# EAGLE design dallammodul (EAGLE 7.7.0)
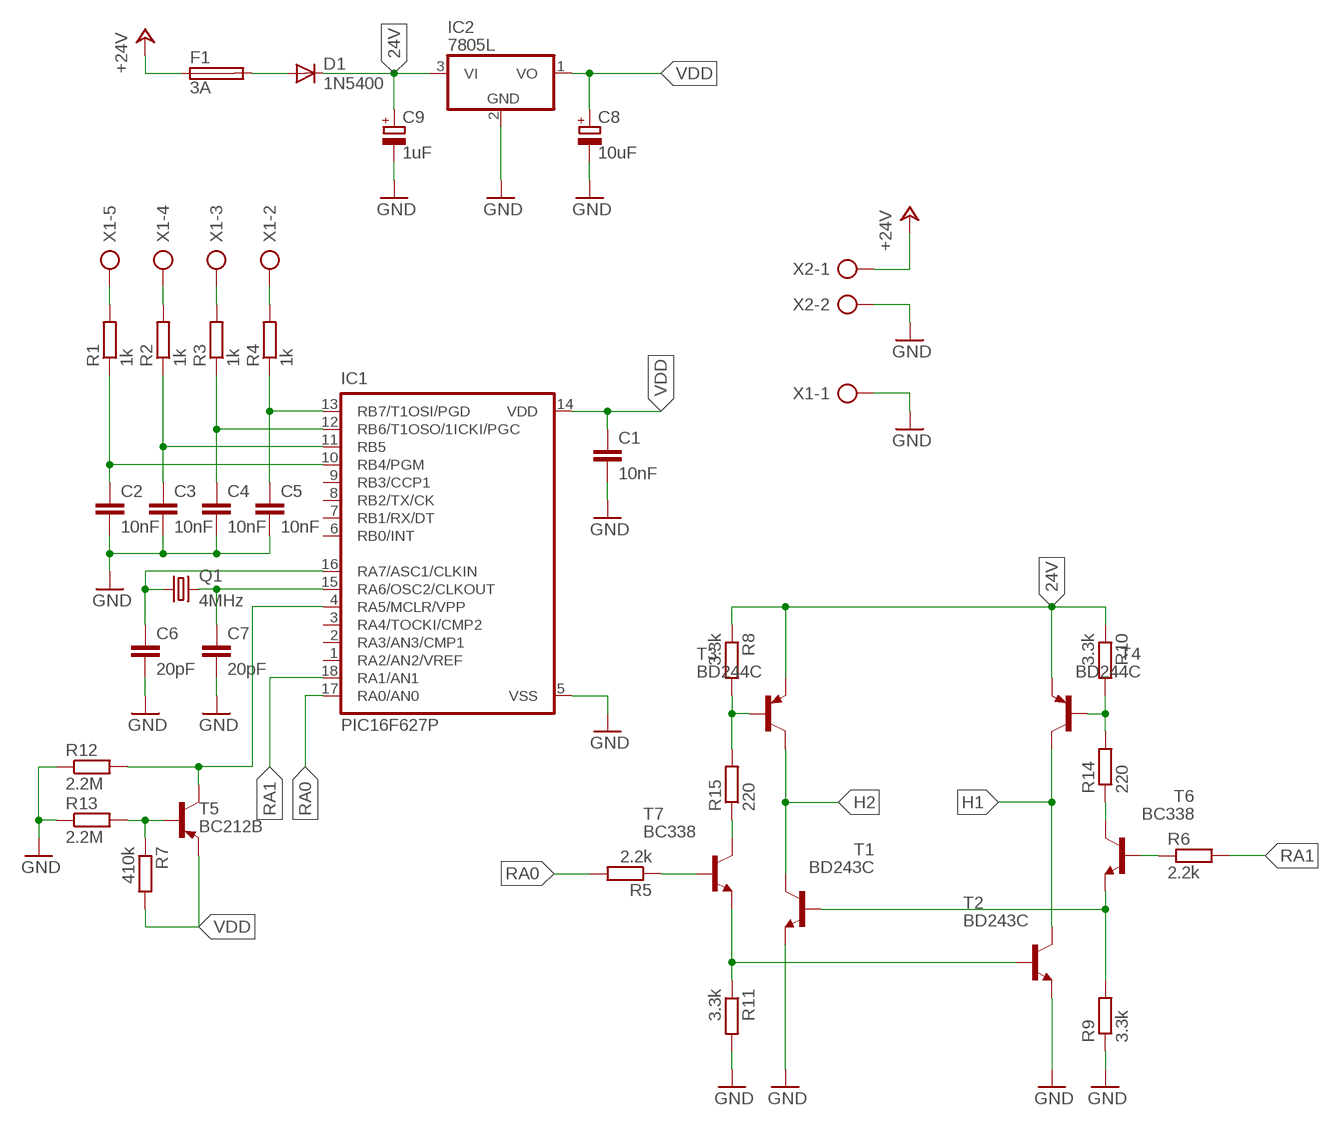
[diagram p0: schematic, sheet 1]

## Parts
C1  10nF  C-EU050-024X044  [C050-024X044]
C2  10nF  C-EU050-024X044  [C050-024X044]
C3  10nF  C-EU050-024X044  [C050-024X044]
C4  10nF  C-EU050-024X044  [C050-024X044]
C5  10nF  C-EU050-024X044  [C050-024X044]
C6  20pF  C-EU050-024X044  [C050-024X044]
C7  20pF  C-EU050-024X044  [C050-024X044]
C8  10uF  CPOL-EUE2-5  [E2-5]
C9  1uF  CPOL-EUE2-5  [E2-5]
D1  1N5400  [DO201-15]
F1  3A  GSH15  [GSH15]
IC1  PIC16F627P  [DIL18]
IC2  7805L  [TO92]
Q1  4MHz  CRYSTALHC18U-V  [HC18U-V]
R1  1k  R-EU_0207/10  [0207/10]
R2  1k  R-EU_0207/10  [0207/10]
R3  1k  R-EU_0207/10  [0207/10]
R4  1k  R-EU_0207/10  [0207/10]
R5  2.2k  R-EU_0207/10  [0207/10]
R6  2.2k  R-EU_0207/10  [0207/10]
R7  410k  R-EU_0207/10  [0207/10]
R8  3.3k  R-EU_0207/10  [0207/10]
R9  3.3k  R-EU_0207/10  [0207/10]
R10  3.3k  R-EU_0207/10  [0207/10]
R11  3.3k  R-EU_0207/10  [0207/10]
R12  2.2M  R-EU_0309/10  [0309/10]
R13  2.2M  R-EU_0309/10  [0309/10]
R14  220  R-EU_0411/15  [0411/15]
R15  220  R-EU_0411/15  [0411/15]
T1  BD243C  -NPN-TO220V  [TO220V]
T2  BD243C  -NPN-TO220V  [TO220V]
T3  BD244C  -PNP-TO220V  [TO220V]
T4  BD244C  -PNP-TO220V  [TO220V]
T5  BC212B  -PNP-TO92L  [TO92L]
T6  BC338  -NPN-TO92L  [TO92L]
T7  BC338  -NPN-TO92L  [TO92L]
X1  AK300/5  [AK300/5]
X2  AK300/2  [AK300/2]

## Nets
24V: C9.+ D1.C IC2.3(VI) R8.1 R10.1 T3.3(E) T4.3(E)
+24V: F1.1 X2.1
GND: C1.2 C2.2 C3.2 C4.2 C5.2 C6.2 C7.2 C8.- C9.- IC1.5(VSS) IC2.2(GND) R9.1 R11.2 R12.1 R13.1 T1.3(E) T2.3(E) X1.1 X2.2
H1: T2.2(C) T4.2(C)
H2: T1.2(C) T3.2(C)
N$1: C6.1 IC1.16(RA7/ASC1/CLKIN) Q1.1
N$2: C7.1 IC1.15(RA6/OSC2/CLKOUT) Q1.2
N$3: C2.1 IC1.10(RB4/PGM) R1.1
N$4: C3.1 IC1.11(RB5) R2.1
N$5: R5.1 T7.2(B)
N$6: C4.1 IC1.12(RB6/T1OSO/1ICKI/PGC) R3.1
N$7: C5.1 IC1.13(RB7/T1OSI/PGD) R4.1
N$8: R4.2 X1.2
N$9: R3.2 X1.3
N$10: R2.2 X1.4
N$11: R1.2 X1.5
N$14: D1.A F1.2
N$15: R8.2 R15.2 T3.1(B)
N$16: R10.2 R14.2 T4.1(B)
N$17: R7.1 R13.2 T5.2(B)
N$18: R15.1 T7.3(C)
N$19: R6.1 T6.2(B)
N$20: R11.1 T2.1(B) T7.1(E)
N$22: R9.2 T1.1(B) T6.1(E)
N$23: R14.1 T6.3(C)
RA0: IC1.17(RA0/AN0) R5.2
RA1: IC1.18(RA1/AN1) R6.2
RA5: IC1.4(RA5/MCLR/VPP) R12.2 T5.3(C)
VDD: C1.1 C8.+ IC1.14(VDD) IC2.1(VO) R7.2 T5.1(E)
Unconnected: IC1.1(RA2/AN2/VREF) IC1.2(RA3/AN3/CMP1) IC1.3(RA4/TOCKI/CMP2) IC1.6(RB0/INT) IC1.7(RB1/RX/DT) IC1.8(RB2/TX/CK) IC1.9(RB3/CCP1)

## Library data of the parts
C1-C7 = rcl:C-EU: CAPACITOR, European symbol
C8 C9 = rcl:CPOL-EU: POLARIZED CAPACITOR, European symbol
D1 = diode:1N5400: DIODE
F1 = fuse:GSH15: FUSE HOLDER; MPN: 64900001039; OC_FARNELL: 1271673; OC_NEWARK: 02P0318
IC1 = microchip:PIC16*F62: FLASH-Based 8-Bit CMOS Microcontroller Source: http://ww1.microchip.com/downloads/en/DeviceDoc/40300C.pdf; MF: MICROCHIP; MPN: PIC16F627-20I/P; OC_FARNELL: 1084298; OC_NEWARK: 23C4967
IC2 = 78:78*: Positive VOLTAGE REGULATOR Source: http://cache.national.com/ds/LM/LM78L05.pdf http://www.fairchildsemi.com/ds/LM/LM7805.pdf
Q1 = crystal:CRYSTAL: CRYSTAL; OC_FARNELL: unknown; OC_NEWARK: unknown
R1-R15 = rcl:R-EU_: RESISTOR, European symbol
T1 T2 T6 T7 = transistor:*-NPN-: NPN Transistror BF959 corrected 2008.03.06
T3-T5 = transistor:*-PNP-: PNP Transistror
X1 = con-ptr500:AK300/5: CONNECTOR; OC_FARNELL: unknown; OC_NEWARK: unknown
X2 = con-ptr500:AK300/2: CONNECTOR; OC_FARNELL: unknown; OC_NEWARK: unknown

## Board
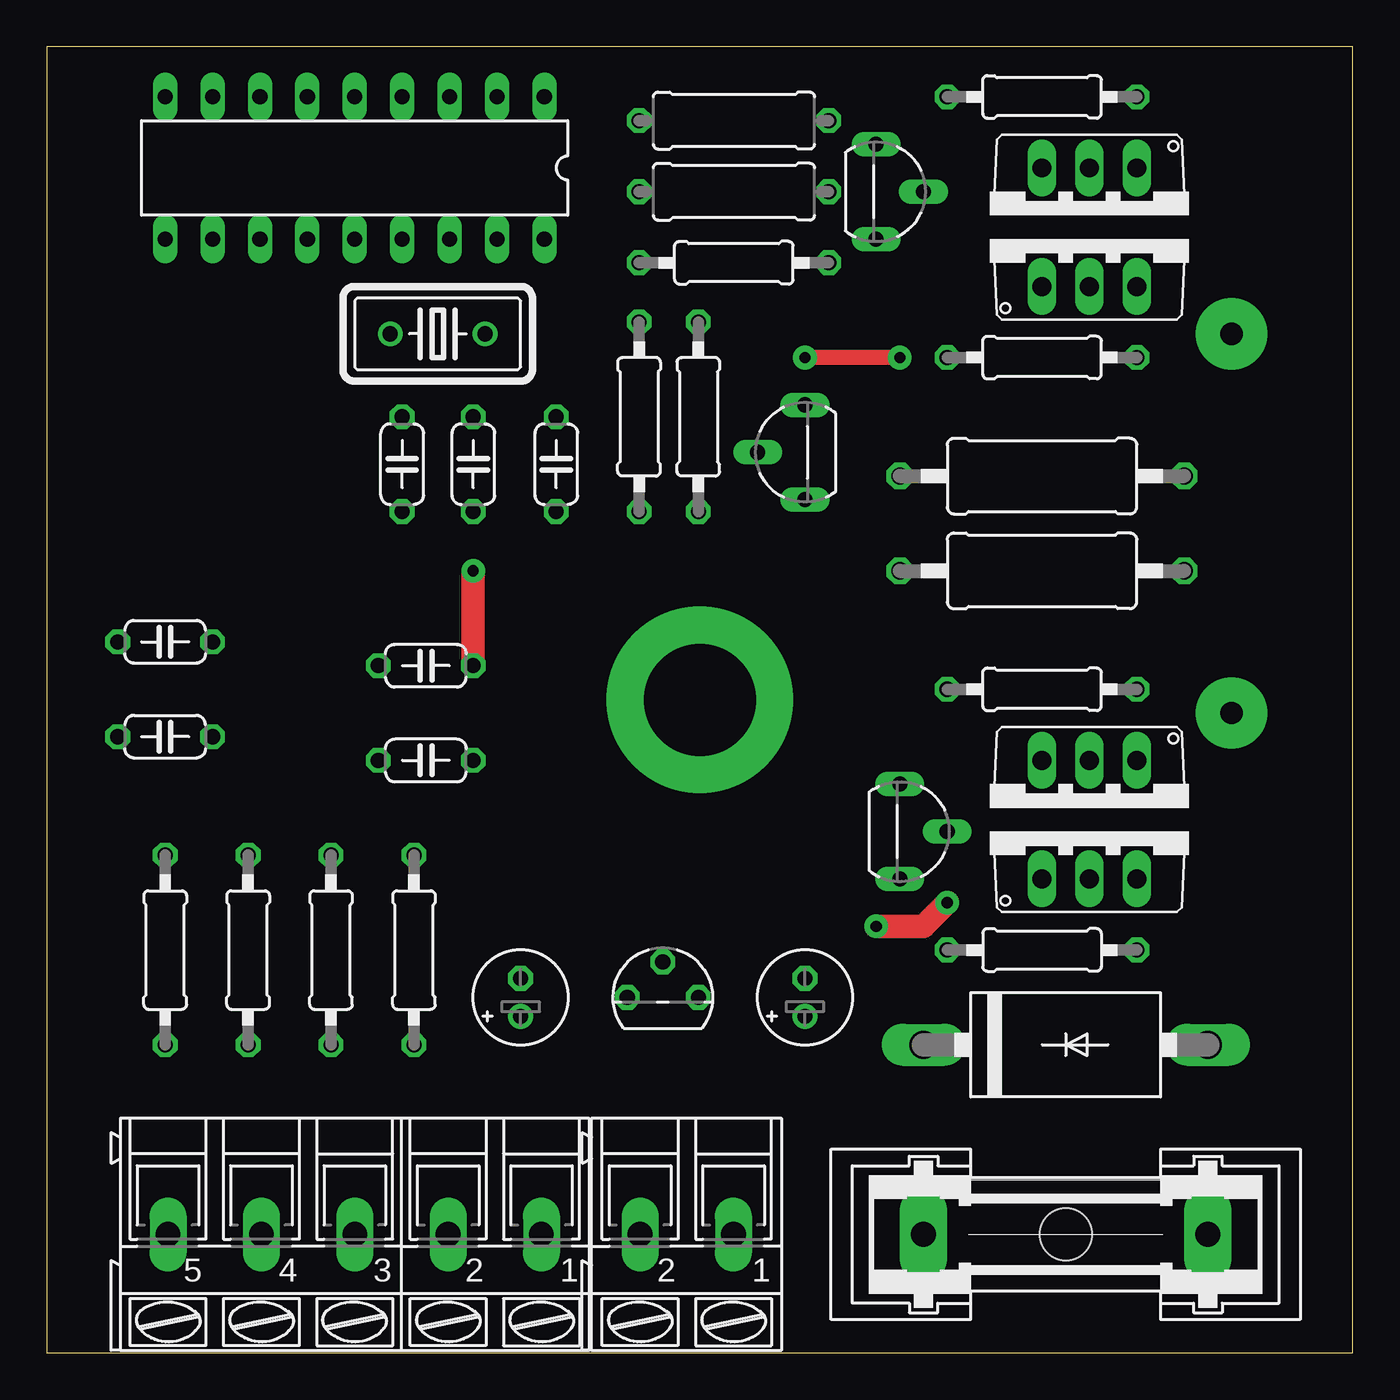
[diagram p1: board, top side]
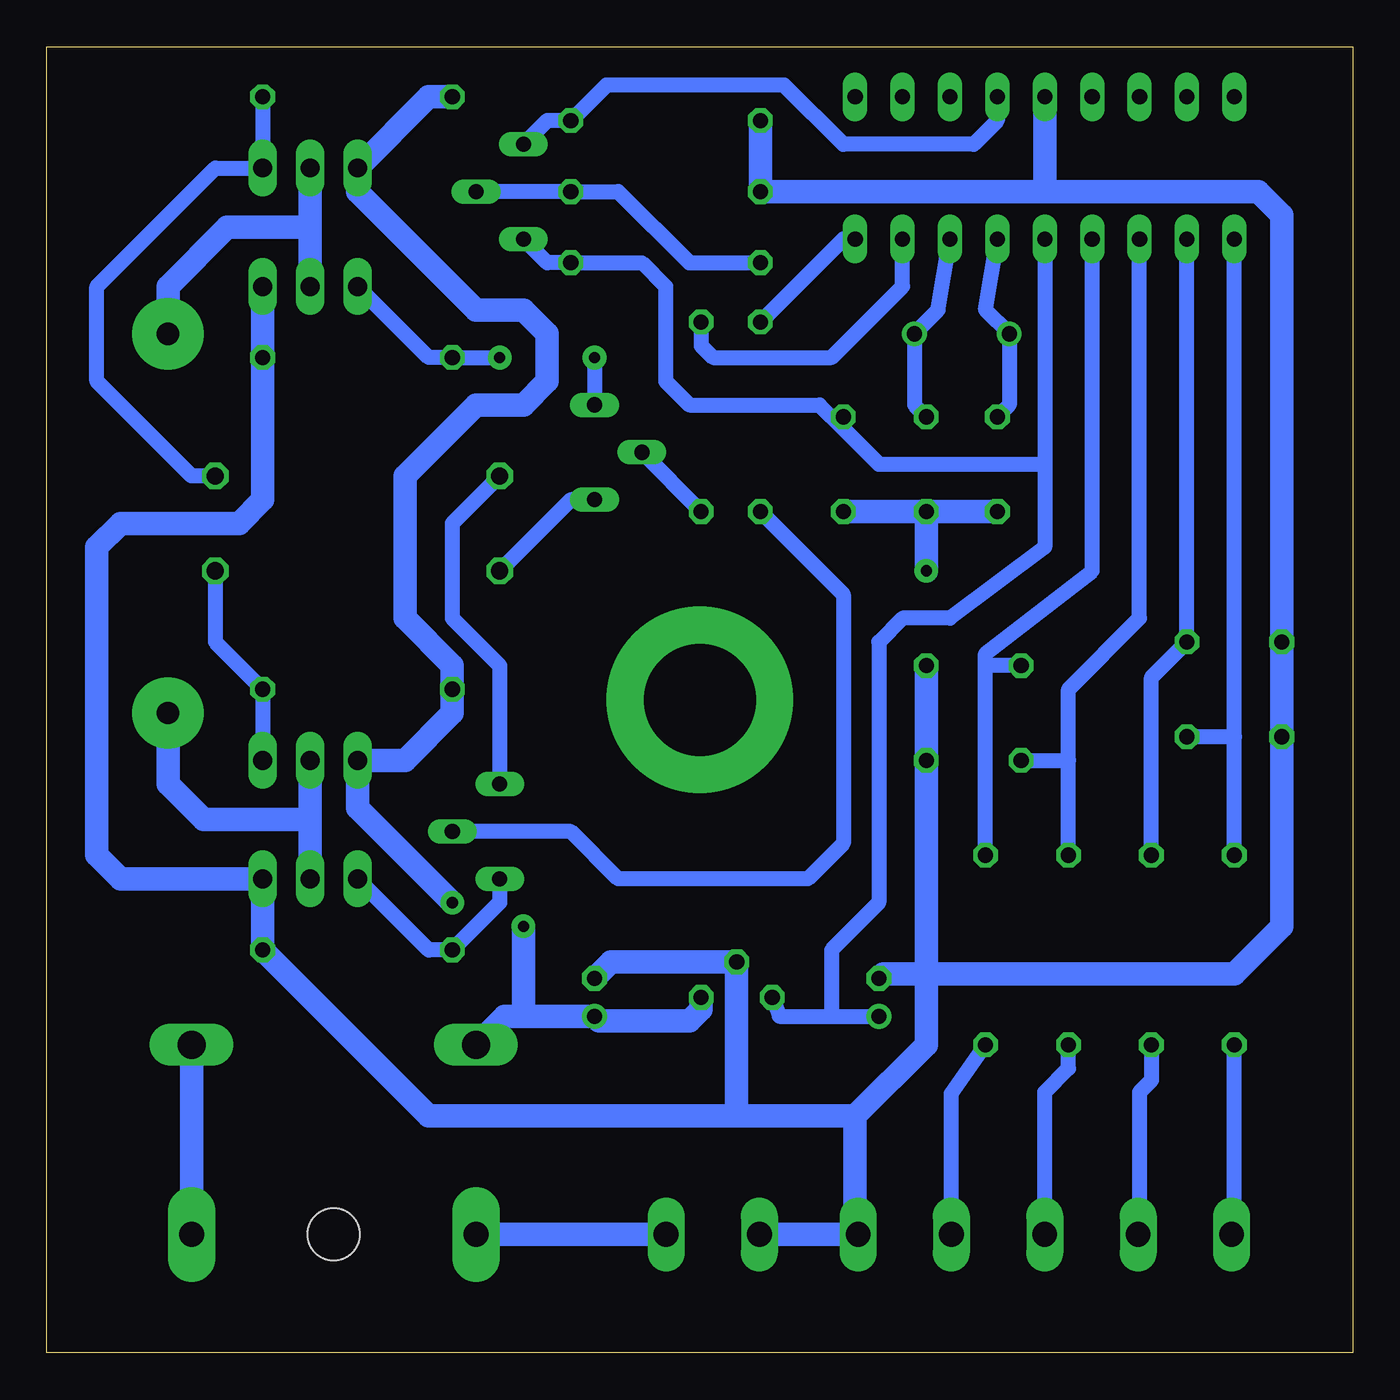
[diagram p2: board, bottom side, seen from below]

Size 70 x 70 mm. Coordinates in mm from the lower left corner, seen from the top.
Outline: 0,0 70,0 70,70 0,70 0,0
Copper layers (1*16): Top 0.035mm / dielectric 1.5mm / Bottom 0.035mm
Design rules "dirt_cheap_dirty_boards.v1": minimum track width 5mil, minimum drill 12mil, track to track 5mil, track to pad 5mil, pad to pad 5mil, via to via 5mil, smd to smd 0mil, copper to edge 10mil, drill to drill 10mil, minimum pad ring 10mil, minimum via ring 6mil, stop-mask expansion 2mil, vias tented up to drill 25mil, thermal gap 10mil

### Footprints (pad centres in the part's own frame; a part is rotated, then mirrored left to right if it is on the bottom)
C050-024X044 = drill 0.813 octagon: 1 -2.54,0; 2 2.54,0
E2-5 = drill 0.813 pad 1.27: + -1.016,0 | drill 0.813 pad 1.27 octagon: - 1.016,0
DO201-15 = drill 1.499 long: A 7.62,0; C -7.62,0
GSH15 = drill 1.321 pad 2.54 long: 1 -7.62,0; 2 7.62,0 | hole 2.794: 0,0
DIL18 = drill 0.813 long: 1 -10.16,-3.81; 2 -7.62,-3.81; 3 -5.08,-3.81; 4 -2.54,-3.81; 5 0,-3.81; 6 2.54,-3.81; 7 5.08,-3.81; 8 7.62,-3.81; 9 10.16,-3.81; 10 10.16,3.81; 11 7.62,3.81; 12 5.08,3.81; 13 2.54,3.81; 14 0,3.81; 15 -2.54,3.81; 16 -5.08,3.81; 17 -7.62,3.81; 18 -10.16,3.81
TO92 = drill 0.813 octagon: 1 -1.905,0; 2 0,1.905; 3 1.905,0
HC18U-V = drill 0.813: 1 -2.54,0; 2 2.54,0
0207/10 = drill 0.813 octagon: 1 -5.08,0; 2 5.08,0
0309/10 = drill 0.813 octagon: 1 -5.08,0; 2 5.08,0
0411/15 = drill 0.914 octagon: 1 -7.62,0; 2 7.62,0
TO220V = drill 1.016 long: 1 -2.54,-2.54; 2 0,-2.54; 3 2.54,-2.54
TO92L = drill 0.813 long: 1 0,-2.54; 2 2.54,0; 3 0,2.54
AK300/5 = drill 1.321 long: 1 -10.008,0; 2 -5.004,0; 3 0,0; 4 5.004,0; 5 10.008,0
AK300/2 = drill 1.321 long: 1 -2.515,0; 2 2.489,0

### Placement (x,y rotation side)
C1  27.3,47.62 270 top
C2  6.35,33.02 180 top
C3  6.35,38.1 180 top
C4  20.32,31.75 0 top
C5  20.32,36.83 0 top
C6  22.86,47.62 270 top
C7  19.05,47.62 270 top
C8  25.4,19.05 90 top
C9  40.64,19.05 90 top
D1  54.61,16.51 0 top
F1  54.61,6.35 0 top
IC1  16.51,63.5 180 top
IC2  33.02,19.05 0 top
Q1  20.95,54.61 180 top
R1  6.35,21.59 270 top
R2  10.79,21.59 270 top
R3  15.24,21.59 270 top
R4  19.68,21.59 270 top
R5  34.92,50.16 90 top
R6  31.75,50.16 90 top
R7  36.83,58.42 0 top
R8  53.34,35.56 0 top
R9  53.34,21.59 180 top
R10  53.34,67.31 0 top
R11  53.34,53.34 0 top
R12  36.83,66.04 0 top
R13  36.83,62.23 0 top
R14  53.34,46.99 0 top
R15  53.34,41.91 0 top
T1  55.88,27.94 0 top
T2  55.88,59.69 0 top
T3  55.88,29.21 180 top
T4  55.88,60.96 180 top
T5  44.45,62.23 0 top
T6  45.72,27.94 0 top
T7  40.64,48.26 180 top
X1  16.51,6.35 180 top
X2  34.29,6.35 180 top

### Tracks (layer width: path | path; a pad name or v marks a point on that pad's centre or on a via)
24V  (via drill 0.6 pad 1.27)
  Top 1.27: v44.45,22.86 46.99,22.86 v48.26,24.13
  Bottom 0.813: T4.3 53.34,62.23
  Bottom 1.27: R10.1 49.53,67.31 T4.3 | 53.34,62.23 46.99,55.88 44.45,55.88 43.18,54.61 43.18,52.07 44.45,50.8 46.99,50.8 50.8,46.99 50.8,39.37 48.26,36.83 R8.1 48.26,34.29 50.8,31.75 T3.3 53.34,29.21 v48.26,24.13 | 44.45,18.03 C9.+ 40.39,17.78 35.56,17.78 34.92,18.41 IC2.3 | 44.45,18.03 45.47,18.03 D1.C | v44.45,22.86 44.45,18.03
+24V
  Bottom 1.27: X2.1 F1.1
GND  (via drill 0.6 pad 1.27)
  Top 1.27: C5.2 v22.86,41.91
  Bottom 1.27: C9.- 39.75,20.95 IC2.2 33.02,12.7 | X2.2 X1.1 26.67,6.5 26.67,12.7 | 16.51,62.23 5.08,62.23 3.81,60.96 C3.2 C2.2 3.81,22.86 6.35,20.32 22.86,20.32 | 26.67,12.7 22.86,16.51 22.86,20.32 | 22.86,20.32 C4.2 C5.2 | C8.- 25.15,20.32 22.86,20.32 | v22.86,41.91 C6.2 | C7.2 C6.2 | C6.2 C1.2 | 33.02,12.7 26.67,12.7 | R12.1 R13.1 16.51,62.23 | IC1.5 16.51,62.23 | T2.3 R11.2 58.42,45.72 59.69,44.45 66.04,44.45 67.31,43.18 67.31,26.67 66.04,25.4 T1.3 R9.1 49.53,12.7 33.02,12.7
H1  (via drill 1.2 pad 3.81)
  Bottom 1.27: T4.2 55.88,60.33 | 55.88,60.33 T2.2 | v63.5,54.61 63.5,57.15 60.33,60.33 55.88,60.33
H2  (via drill 1.2 pad 3.81)
  Bottom 1.27: T1.2 55.88,28.57 | 55.88,28.57 T3.2 | v63.5,34.29 63.5,30.48 61.59,28.57 55.88,28.57
N$1
  Bottom 0.813: IC1.16 22.23,55.88 Q1.1 23.5,50.8 C6.1
N$2
  Bottom 0.813: IC1.15 19.68,55.88 Q1.2 18.41,50.8 C7.1
N$3
  Bottom 0.813: R1.1 6.35,33.02 | 6.35,33.02 IC1.10 | C2.1 6.35,33.02
N$4
  Bottom 0.813: R2.1 10.79,36.2 C3.1 IC1.11
N$5
  Bottom 0.813: R5.1 T7.2
N$6
  Bottom 0.813: R3.1 15.24,31.75 | 15.24,31.75 15.24,35.56 11.43,39.37 IC1.12 | C4.1 15.24,31.75
N$7
  Bottom 0.813: R4.1 19.68,36.83 | 19.68,36.83 19.68,37.47 13.97,41.91 IC1.13 | C5.1 19.68,36.83
N$8
  Bottom 0.813: X1.2 21.51,13.89 R4.2
N$9
  Bottom 0.813: X1.3 16.51,13.97 15.24,15.24 R3.2
N$10
  Bottom 0.813: R2.2 10.79,14.61 11.43,13.97 11.43,6.43 X1.4
N$11
  Bottom 0.813: 6.35,6.35 R1.2
  Bottom 1.016: X1.5 6.35,6.35
N$12  (via drill 6 pad 10)
  other vias: 35,35
N$14
  Bottom 1.27: F1.2 D1.A
N$15
  Bottom 0.813: R15.2 60.96,38.1 R8.2 T3.1
N$16
  Bottom 0.813: R14.2 62.23,46.99 67.31,52.07 67.31,57.15 60.96,63.5 T4.1 R10.2
N$17
  Bottom 0.813: R7.1 35.56,58.42 39.37,62.23 R13.2 T5.2
N$18
  Bottom 0.813: T7.3 41.91,45.72 R15.1
N$19
  Bottom 0.813: R6.1 27.3,40.64 27.3,27.3 29.21,25.4 39.37,25.4 41.91,27.94 T6.2
N$20  (via drill 0.6 pad 1.27)
  Top 0.813: v45.72,53.34 v40.64,53.34
  Bottom 0.813: v45.72,53.34 R11.1 49.53,53.34 T2.1 | v40.64,53.34 T7.1
N$22
  Bottom 0.813: T6.1 45.72,24.13 R9.2 49.53,21.59 T1.1
N$23
  Bottom 0.813: R14.1 48.26,44.45 48.26,39.37 45.72,36.83 T6.3
RA0
  Bottom 0.813: R5.2 34.92,53.98 34.29,53.34 27.94,53.34 24.13,57.15 IC1.17
RA1
  Bottom 0.813: IC1.18 27.3,59.69 R6.2
RA5
  Bottom 0.813: IC1.4 19.05,66.04 20.32,64.77 27.3,64.77 30.48,67.94 40.01,67.94 R12.2 43.18,66.04 T5.3
VDD
  Bottom 0.813: IC2.1 30.73,18.03 27.94,18.03 | 27.94,18.03 C8.+ | IC1.14 16.51,47.62 | 16.51,47.62 16.51,43.18 21.59,39.37 24.13,39.37 25.4,38.1 25.4,24.13 27.94,21.59 27.94,18.03 | C1.1 27.3,49.53 | 27.3,49.53 25.4,47.62 16.51,47.62 | 27.3,49.53 28.57,50.8 35.56,50.8 36.83,52.07 36.83,57.15 38.1,58.42 R7.2 43.18,58.42 T5.1

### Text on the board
tValues: H | -H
